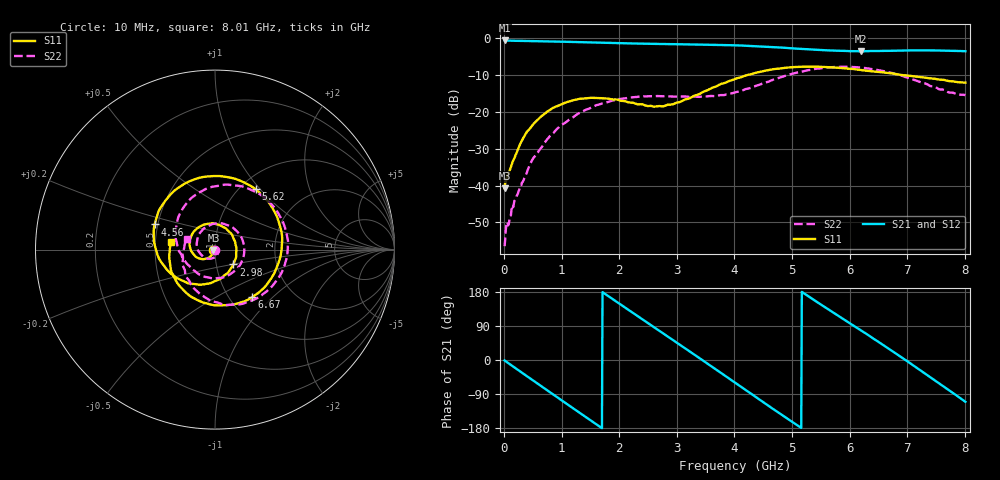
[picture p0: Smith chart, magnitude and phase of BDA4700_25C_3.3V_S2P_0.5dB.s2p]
!Agilent Technologies,E5071B,MY42404982,A.09.10
!Date: Mon Oct 20 18:03:10 2025
!Data & Calibration Information:
!Freq	S11:SOLT2(ON)	S21:SOLT2(ON)	S12:SOLT2(ON)	S22:SOLT2(ON)
# Hz S RI R 50
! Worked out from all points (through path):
!   801 points, 10 MHz to 8.01 GHz, reference 50 ohm
!   highest |S21| = -0.62 dB at 20 MHz (marker M1); lowest = -3.6 dB at 6.2 GHz (marker M2)
!   group delay of S21, straight-line fit = 286 ps
!   lowest |S11| = -40.7 dB at 10 MHz (marker M3), VSWR 1.02, Z = 49.1 - j0.24 ohm
!   |S11| at or under -10 dB: start of sweep to 4.221 GHz; 6.913 GHz to end of sweep
!   |S22| runs from -56.4 to -7.8 dB; largest |S21 - S12| = 0.011
!   S11 on the Smith chart (normalised r, x): 10 MHz: 0.98, -0.00; 2.98 GHz: 1.21, -0.20; 4.56 GHz: 0.48, +0.16; 5.62 GHz: 1.17, +0.95; 6.67 GHz: 1.27, -0.76; 8.01 GHz: 0.60, +0.05
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1e7  -0.00886 -0.00244  0.9304 -0.0199  0.9301 -0.0207  -0.00141 -0.000541
2e7  -0.0101 -0.00424  0.9299 -0.0362  0.9297 -0.0388  -0.00157 0.00101
3.6e8  -0.0271 -0.0395  0.7139 -0.5725  0.714 -0.5725  0.0126 -0.00254
7.2e8  -0.082 -0.0511  0.2058 -0.8807  0.2061 -0.8806  0.00274 -0.0397
1.02e9  -0.1285 -0.014  -0.2836 -0.8484  -0.2837 -0.8486  -0.0484 -0.0478
1.35e9  -0.138 0.0609  -0.7067 -0.5282  -0.7065 -0.5281  -0.0991 0.0109
1.92e9  -0.0237 0.1456  -0.7916 0.3327  -0.792 0.3326  -0.00374 0.1443
2.32e9  0.0771 0.1003  -0.3685 0.7591  -0.3683 0.759  0.1289 0.095
2.68e9  0.1196 0.00893  0.1628 0.8189  0.1615 0.8184  0.1594 -0.0387
2.98e9  0.1027 -0.0826  0.5556 0.6126  0.5547 0.6118  0.0967 -0.1294
3.48e9  -0.0284 -0.1879  0.8139 -0.0589  0.8143 -0.059  -0.0642 -0.1485
4.01e9  -0.2446 -0.1348  0.4035 -0.69  0.4047 -0.689  -0.1757 -0.0526
4.56e9  -0.3363 0.1404  -0.3532 -0.6782  -0.3522 -0.6794  -0.2152 0.132
4.95e9  -0.2042 0.3445  -0.6795 -0.2747  -0.6795 -0.2784  -0.1189 0.297
5.35e9  0.0536 0.4062  -0.6645 0.2234  -0.6661 0.2192  0.1128 0.3569
5.62e9  0.2264 0.3363  -0.4805 0.485  -0.4813 0.4856  0.2778 0.2878
6.2e9  0.3686 -0.0166  0.139 0.6488  0.1482 0.6502  0.3899 -0.0814
6.67e9  0.2059 -0.2657  0.5786 0.3433  0.5795 0.342  0.1833 -0.2911
6.68e9  0.2006 -0.2693  0.5848 0.3333  0.5859 0.3319  0.1775 -0.2933
7.24e9  -0.1179 -0.2713  0.6006 -0.3258  0.6006 -0.3261  -0.1025 -0.2293
7.63e9  -0.2435 -0.1211  0.2327 -0.6347  0.2325 -0.6356  -0.1829 -0.0817
8.01e9  -0.2455 0.0423  -0.2316 -0.6234  -0.2294 -0.6245  -0.1584 0.0593
